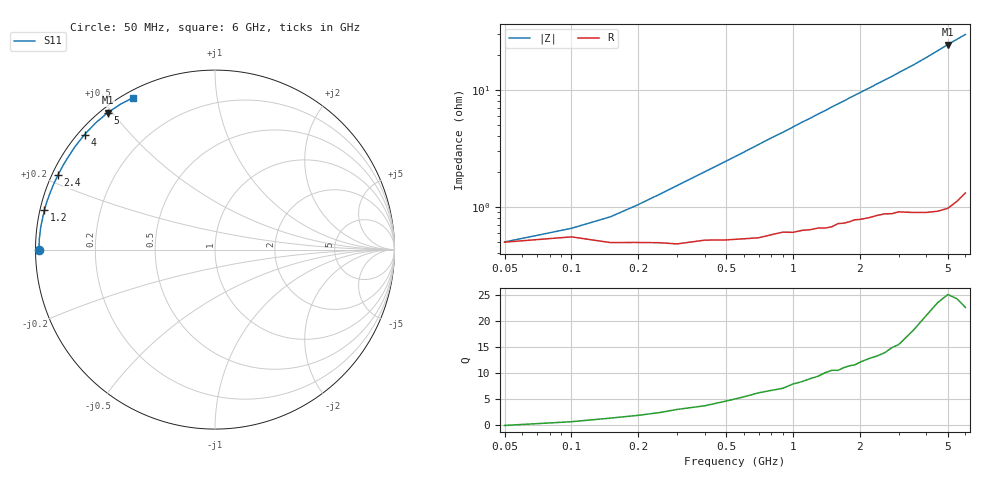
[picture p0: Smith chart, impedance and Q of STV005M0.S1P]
! SIEMENS Discrete & RF Semiconductors
! BA892
! Si PIN Diode in SCD-80
! IF = 5 mA
! S-Parameters:  September  1997
# GHz  S  MA  R  50
!  f  S11
! GHz  MAG  ANG
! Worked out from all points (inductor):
!   34 points, 50 MHz to 6 GHz, reference 50 ohm
!   read as one part to ground: L = 765 pH near 400 MHz
!   highest Q = 24.3 at 5 GHz (marker M1), where L = 776 pH
!   S11 on the Smith chart (normalised r, x): 50 MHz: 0.01, -0.00; 1.2 GHz: 0.01, +0.11; 2.4 GHz: 0.02, +0.22; 4 GHz: 0.02, +0.38; 5 GHz: 0.02, +0.49; 6 GHz: 0.03, +0.59
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0.05  0.9803 -179.9
0.1  0.9781 179.2
0.15  0.9804 178.5
0.3  0.981 176.7
0.6  0.979 173.4
0.7  0.9786 172.3
0.8  0.9773 171.2
0.9  0.9762 170.2
1  0.9763 169.1
1.1  0.9755 168.0
1.2  0.9752 167.0
1.3  0.9744 165.9
1.4  0.9745 164.9
1.5  0.9739 163.8
1.6  0.9723 162.8
1.7  0.9722 161.8
1.8  0.9715 160.7
2.2  0.9696 156.7
2.4  0.9684 154.7
2.6  0.9677 152.7
2.8  0.9678 150.8
3  0.967 148.7
3.5  0.9682 143.8
4  0.9692 138.6
4.5  0.9696 133.3
5  0.9691 128.0
5.5  0.9661 123.1
6  0.962 118.5
